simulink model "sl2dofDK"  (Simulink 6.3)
settings: Solver=ode45  SolverMode=SingleTasking  StartTime=0.0  StopTime=dkt2  RelTol=1e-2  AbsTol=1e-6
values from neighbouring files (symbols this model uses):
  a0 = a0tmp    (= 0)    [gsdata.m]    (also in runme.m = 1; per.m = a0+das0*sin(oma0*t))
  a1 = a1tmp    (= 0)    [gsdata.m]    (also in runme.m = 2; getcfactors.m = poly(aRoots1*f)*a(max(size(a))-deg(a)+1); per.m = a1+das1*sin(oma1*t))
  a2 = a2tmp    (= 0)    [gsdata.m]    (also in runme.m = 1; getcfactors.m = poly(maxroot(1:maxj)*f); per.m = a2+das2*sin(oma2*t))
  a3 = a3tmp    (= 0)    [gsdata.m]    (also in runme.m; per.m = a3+das3*sin(oma3*t))
  a4 = a4tmp    (= 0)    [gsdata.m]    (also in runme.m)
  b0 = b0tmp    (= 0)    [gsdata.m]    (also in runme.m = 2; per.m = b0+dbs0*sin(omb0*t))
  b1 = b1tmp    (= 0)    [gsdata.m]    (also in runme.m; per.m = b1+dbs1*sin(omb1*t))
  b2 = b2tmp    (= 0)    [gsdata.m]    (also in runme.m; per.m = b2+dbs2*sin(omb2*t))
  b3 = b3tmp    (= 0)    [gsdata.m]    (also in runme.m; per.m = b3+dbs3*sin(omb3*t))
  b_kdk1fw = [b_kdk1(degb_kdk1)]    [Getkdkdp.m]
  dkdst2 = 120    [runme.m]    (also in dkdata.m = 0)
  dkdsv2 = 0.2    [runme.m]    (also in dkdata.m = 0)
  dkrst2 = 1    [runme.m]    (also in dkdata.m = 0)
  dkrsv2 = 1    [runme.m]    (also in dkdata.m = 0)
  dkt2 = 200    [runme.m]    (also in dkdata.m = 0)
  m0dk = 1    [runme.m]    (also in dkccpe.m = 0)
  m1dk = 0    [runme.m]    (also in dkccpe.m)
  m2dk = 0    [runme.m]    (also in dkccpe.m)
  m3dk = 0    [runme.m]    (also in dkccpe.m)
  r0dk = 1    [runme.m]    (also in dkccpe.m = 0)
  r1dk = 0    [runme.m]    (also in dkccpe.m)
  r2dk = 0    [runme.m]    (also in dkccpe.m)
  r3dk = 0    [runme.m]    (also in dkccpe.m)
  Td = Tdtmp    (= 0)    [gsdata.m]    (also in runme.m = 4)
undefined symbols (not defined in the file or in its folder): a_kdk1, a_kdk2, b_kdk1, b_kdk2

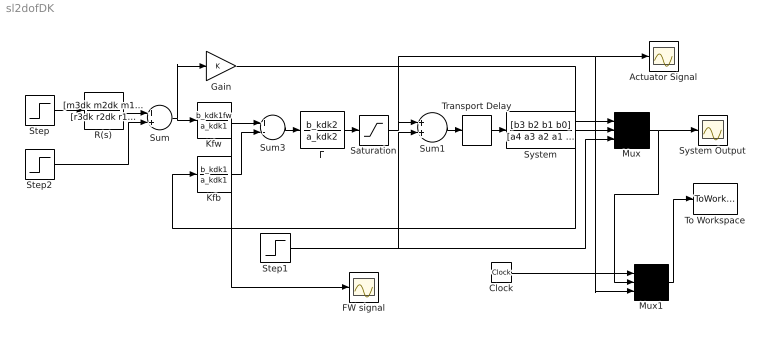
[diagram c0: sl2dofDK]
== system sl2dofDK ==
  Actuator Signal : Scope
  Clock : Clock
  F : TransferFcn  Numerator=b_kdk2  Denominator=a_kdk2
  FW signal : Scope
  Gain : Gain
  Kfb : TransferFcn  Numerator=b_kdk1  Denominator=a_kdk1
  Kfw : TransferFcn  Numerator=b_kdk1fw  Denominator=a_kdk1
  Mux : Mux  Inputs=3
  Mux1 : Mux  Inputs=3
  R(s) : TransferFcn  Numerator=[m3dk m2dk m1dk m0dk]  Denominator=[r3dk r2dk r1dk r0dk]
  Saturation : Saturate  UpperLimit=10  LowerLimit=-10
  Step : Step  Time=dkrst2  After=dkrsv2  SampleTime=0
  Step1 : Step  Time=400  After=0  SampleTime=0
  Step2 : Step  Time=dkdst2  After=dkdsv2  SampleTime=0
  Sum : Sum
  Sum1 : Sum
  Sum3 : Sum  Inputs=+-
  System : TransferFcn  Numerator=[b3 b2 b1 b0]  Denominator=[a4 a3 a2 a1 a0]
  System Output : Scope
  To Workspace : ToWorkspace  VariableName=o2  SampleTime=dkt2/500  SaveFormat=Array
  Transport Delay : TransportDelay  DelayTime=Td  BufferSize=5000
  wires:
  Gain/1 -> Mux/1
  Sum1/1 -> Transport Delay/1
  Step1/1 -> Sum1/2, Mux/3
  Mux/1 -> System Output/1, Mux1/2
  Mux1/1 -> To Workspace/1
  Clock/1 -> Mux1/1
  Transport Delay/1 -> System/1
  System/1 -> Mux/2, Kfb/1
  Kfw/1 -> Sum3/1, FW signal/1
  Kfb/1 -> Sum3/2
  Saturation/1 -> Sum1/1, Actuator Signal/1, Mux1/3
  F/1 -> Saturation/1
  Sum3/1 -> F/1
  Step/1 -> R(s)/1
  R(s)/1 -> Sum/1
  Step2/1 -> Sum/2
  Sum/1 -> Kfw/1, Gain/1
